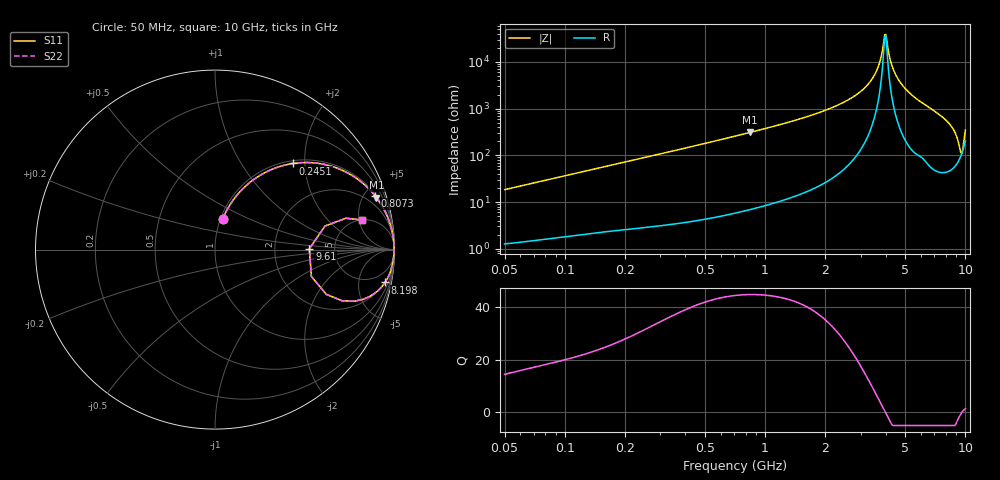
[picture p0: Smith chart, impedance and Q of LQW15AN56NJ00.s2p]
!Murata Part Number: LQW15AN56NJ00
!These Parameters are Measured in Series Mode Connection
!  o--[Z]--o
!Port1  Port2
!  o-------o
!Freq. Start=50[MHz] Stop=10[GHz], 401[Steps]
# Hz S RI R 50
!Freq.(Hz)	S 11(Real)	S 11(Imag)	S 21(Real)	S 21(Imag)	S 12(Real)	S 12(Imag)	S 22(Real)	S 22(Imag)
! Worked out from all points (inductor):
!   401 points, 50 MHz to 10 GHz, reference 50 ohm
!   read as one part in series: L = 58.2 nH near 51.34 MHz
!   highest Q = 44.8 at 840 MHz (marker M1), where L = 58.4 nH
!   self-resonance near 3.957 GHz
!   S11 on the Smith chart (normalised r, x): 50 MHz: 1.03, +0.37; 245.1 MHz: 1.06, +1.75; 807.3 MHz: 1.13, +5.91; 8.198 GHz: 2, -10; 9.61 GHz: 3.22, +0.05; 10 GHz: 5.07, +5.59
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5e7  0.0439 0.1733  0.9561 -0.1733  0.9561 -0.1733  0.0439 0.1733
1.214486e8  0.1725 0.3555  0.8275 -0.3555  0.8275 -0.3555  0.1725 0.3555
2.450637e8  0.4361 0.4801  0.5639 -0.4801  0.5639 -0.4801  0.4361 0.4801
2.949953e8  0.5253 0.485  0.4747 -0.485  0.4747 -0.485  0.5253 0.485
7.071068e8  0.8629 0.3329  0.1371 -0.3329  0.1371 -0.3329  0.8629 0.3329
8.07255e8  0.892 0.2994  0.108 -0.2994  0.108 -0.2994  0.892 0.2994
8.399791e8  0.8997 0.2894  0.1003 -0.2894  0.1003 -0.2894  0.8997 0.2894
1.717543e9  0.9783 0.1335  0.0217 -0.1335  0.0217 -0.1335  0.9783 0.1335
2.488741e9  0.9923 0.0711  0.00774 -0.0711  0.00774 -0.0711  0.9923 0.0711
3.158828e9  0.9964 0.0348  0.00361 -0.0348  0.00361 -0.0348  0.9964 0.0348
3.606216e9  0.9974 0.0151  0.00258 -0.0151  0.00258 -0.0151  0.9974 0.0151
3.956578e9  0.9976 0.00107  0.00239 -0.00107  0.00239 -0.00107  0.9976 0.00107
4.062795e9  0.9976 -0.00299  0.00242 0.00299  0.00242 0.00299  0.9976 -0.00299
4.171863e9  0.9975 -0.00708  0.00249 0.00708  0.00249 0.00708  0.9975 -0.00708
4.457516e9  0.9972 -0.0175  0.00284 0.0175  0.00284 0.0175  0.9972 -0.0175
4.955797e9  0.9959 -0.0351  0.00407 0.0351  0.00407 0.0351  0.9959 -0.0351
8.198065e9  0.9476 -0.1829  0.0524 0.1829  0.0524 0.1829  0.9476 -0.1829
8.759398e9  0.8884 -0.2444  0.1116 0.2444  0.1116 0.2444  0.8884 -0.2444
9.114482e9  0.7787 -0.2875  0.2213 0.2875  0.2213 0.2875  0.7787 -0.2875
9.359165e9  0.6197 -0.2491  0.3803 0.2491  0.3803 0.2491  0.6197 -0.2491
9.610418e9  0.5257 0.00508  0.4743 -0.00508  0.4743 -0.00508  0.5257 0.00508
1e10  0.8216 0.1641  0.1784 -0.1641  0.1784 -0.1641  0.8216 0.1641
